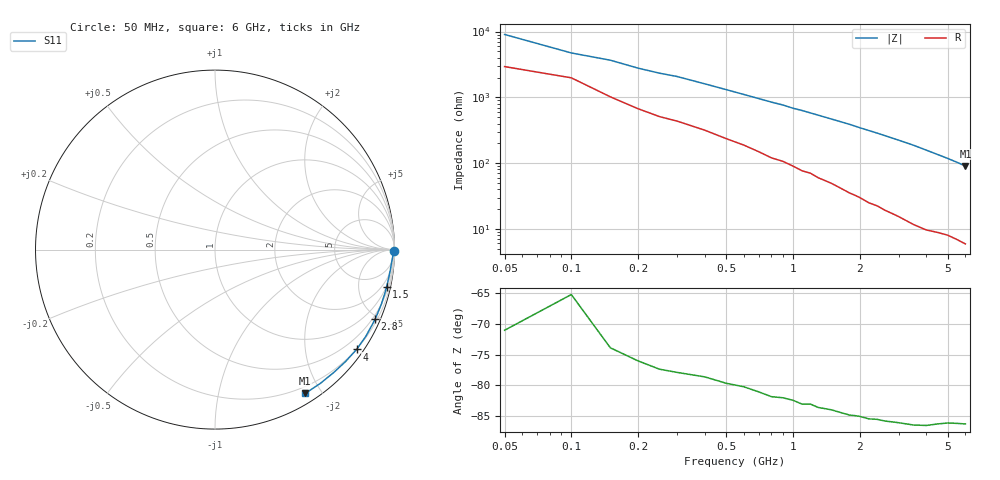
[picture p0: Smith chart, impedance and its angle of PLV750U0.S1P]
! Infineon Technologies  Discrete & RF Semiconductors
! BAR 64-04W /-05W /-06W
! Si PIN Diode in SOT323
! VR = 0.75 V
! S-Parameters:  October  2008
# GHz  S  MA  R  50
!  f  S11
! GHz  MAG  ANG
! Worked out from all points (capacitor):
!   34 points, 50 MHz to 6 GHz, reference 50 ohm
!   read as one part to ground: C = 370 fF near 50 MHz
!   lowest |Z| = 90.3 ohm at 6 GHz (marker M1)
!   S11 on the Smith chart (normalised r, x): 50 MHz: open; 1.5 GHz: 0.98, -9.26; 2.8 GHz: 0.34, -4.81; 4 GHz: 0.19, -3.14; 6 GHz: 0.12, -1.80
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0.05  0.9964 -0.6
0.1  0.9912 -1.1
0.15  0.9925 -1.5
0.2  0.9913 -2.0
0.25  0.9907 -2.4
0.3  0.9899 -2.7
0.6  0.9848 -5.1
0.8  0.9834 -6.7
0.9  0.9821 -7.4
1  0.9809 -8.3
1.1  0.9811 -9.0
1.2  0.9794 -9.8
1.3  0.9795 -10.6
1.5  0.978 -12.2
1.6  0.9777 -13.0
1.8  0.9774 -14.6
2  0.9757 -16.4
2.2  0.9755 -18.1
2.4  0.9737 -19.8
2.6  0.9732 -21.6
2.8  0.972 -23.4
3  0.971 -25.2
3.5  0.9693 -29.9
4  0.9653 -35.2
4.5  0.9582 -40.6
5  0.9521 -46.0
5.5  0.9486 -51.8
6  0.946 -57.9
